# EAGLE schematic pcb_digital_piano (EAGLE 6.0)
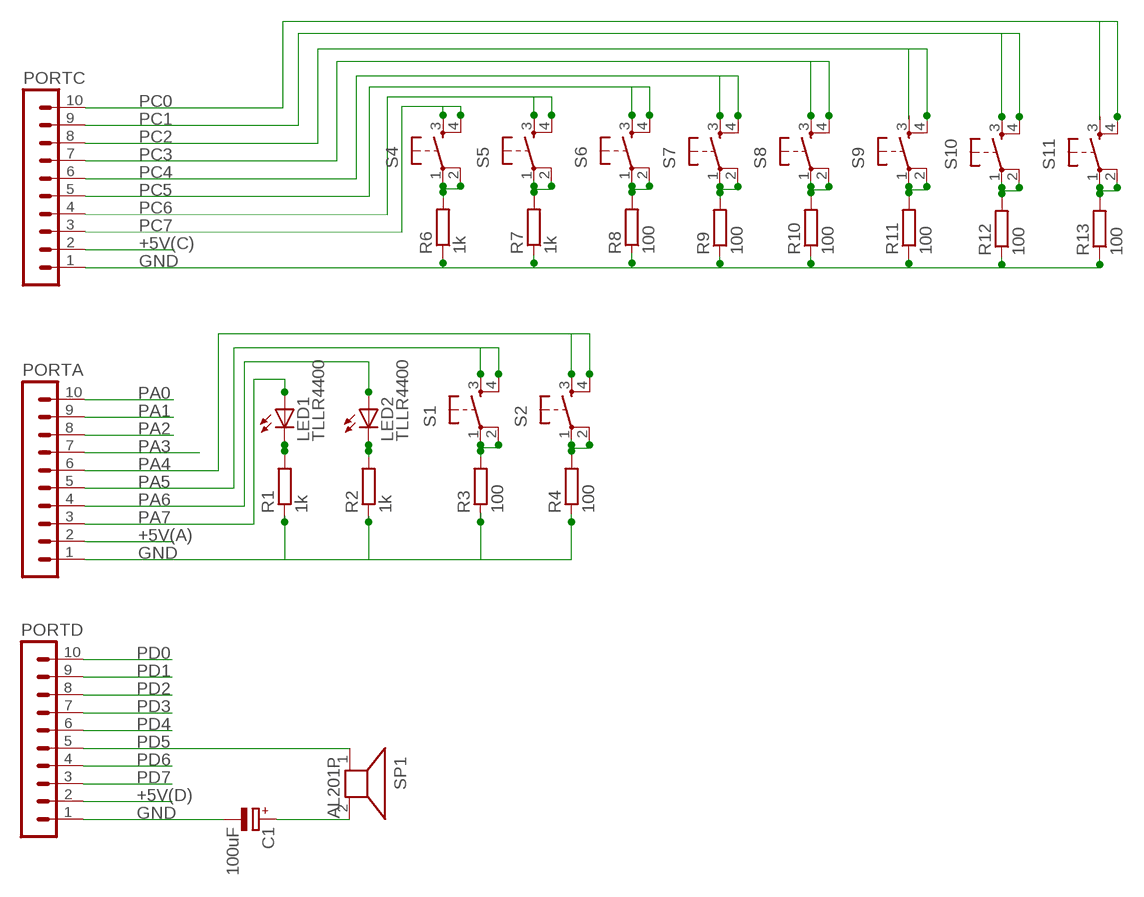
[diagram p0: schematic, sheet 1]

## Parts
C1  100uF  CPOL-EUE2.5-5  [E2,5-5]
LED1  TLLR4400  [LED3MM]
LED2  TLLR4400  [LED3MM]
PORTA  MA10-1W  [MA10-1W]
PORTC  MA10-1W  [MA10-1W]
PORTD  MA10-1W  [MA10-1W]
R1  1k  R-EU_0204/7  [0204/7]
R2  1k  R-EU_0204/7  [0204/7]
R3  100  R-EU_0204/7  [0204/7]
R4  100  R-EU_0204/7  [0204/7]
R6  1k  R-EU_0204/7  [0204/7]
R7  1k  R-EU_0204/7  [0204/7]
R8  100  R-EU_0204/7  [0204/7]
R9  100  R-EU_0204/7  [0204/7]
R10  100  R-EU_0204/7  [0204/7]
R11  100  R-EU_0204/7  [0204/7]
R12  100  R-EU_0204/7  [0204/7]
R13  100  R-EU_0204/7  [0204/7]
S1  TAC_SWITCHPTH  [TACTILE-PTH]
S2  TAC_SWITCHPTH  [TACTILE-PTH]
S4  TAC_SWITCHPTH  [TACTILE-PTH]
S5  TAC_SWITCHPTH  [TACTILE-PTH]
S6  TAC_SWITCHPTH  [TACTILE-PTH]
S7  TAC_SWITCHPTH  [TACTILE-PTH]
S8  TAC_SWITCHPTH  [TACTILE-PTH]
S9  TAC_SWITCHPTH  [TACTILE-PTH]
S10  TAC_SWITCHPTH  [TACTILE-PTH]
S11  TAC_SWITCHPTH  [TACTILE-PTH]
SP1  AL201P  [AL201P]

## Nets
+5V(A): PORTA.2
+5V(C): PORTC.2
+5V(D): PORTD.2
GND: C1.- PORTA.1 PORTC.1 PORTD.1 R1.1 R2.1 R3.1 R4.1 R6.1 R7.1 R8.1 R9.1 R10.1 R11.1 R12.1 R13.1
N$1: C1.+ SP1.2
N$2: LED1.K(C) R1.2
N$3: LED2.K(C) R2.2
N$4: R3.2 S1.1 S1.2
N$5: R4.2 S2.1 S2.2
N$8: S1.3
N$9: S2.3
N$10: R6.2 S4.1 S4.2
N$11: R7.2 S5.1 S5.2
N$12: R8.2 S6.1
N$13: S6.2
N$14: R9.2 S7.1 S7.2
N$15: R10.2 S8.1 S8.2
N$16: R11.2 S9.1
N$17: S9.2
N$18: R12.2 S10.1 S10.2
N$19: R13.2 S11.1
N$20: S11.2
N$21: S4.3
N$22: S6.3
N$23: S8.3
N$24: S10.3
PA0: PORTA.10
PA1: PORTA.9
PA2: PORTA.8
PA3: PORTA.7
PA4: PORTA.6 S2.4
PA5: PORTA.5 S1.4
PA6: LED2.A PORTA.4
PA7: LED1.A PORTA.3
PC0: PORTC.10 S11.4
PC1: PORTC.9 S10.4
PC2: PORTC.8 S9.4
PC3: PORTC.7 S8.4
PC4: PORTC.6 S7.3 S7.4
PC5: PORTC.5 S6.4
PC6: PORTC.4 S5.3 S5.4
PC7: PORTC.3 S4.4
PD0: PORTD.10
PD1: PORTD.9
PD2: PORTD.8
PD3: PORTD.7
PD4: PORTD.6
PD5: PORTD.5 SP1.1
PD6: PORTD.4
PD7: PORTD.3
Unconnected: S9.3 S11.3

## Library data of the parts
C1 = resistor:CPOL-EU: POLARIZED CAPACITOR, European symbol
LED1 LED2 = led:TLLR4400: Low Current (2mA) LED 3 mm Tinted Diffused Package color RED; MF: VISHAY SEMICONDUCTOR; OC_FARNELL: 1612437
PORTA PORTC PORTD = con-lstb:MA10-1W: PIN HEADER; OC_FARNELL: unknown; OC_NEWARK: unknown
R1-R4 R6-R13 = resistor:R-EU_: RESISTOR, European symbol
S1 S2 S4-S11 = SparkFun:TAC_SWITCH: Momentary Switch Button commonly used for reset or general input. Spark Fun Electronics SKU : COM-00097
SP1 = buzzer:AL201P: SPEAKER; OC_FARNELL: unknown; OC_NEWARK: unknown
